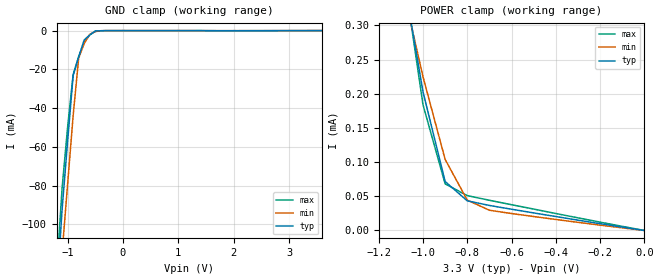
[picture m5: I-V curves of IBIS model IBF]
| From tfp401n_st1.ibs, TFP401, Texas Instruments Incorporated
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|   INPUT  MODEL WITH HYSTERESIS
[Model]   IBF
Model_type   Input
| Signals   STAG
Vinl = 1.08
Vinh = 2.10
| variable   typ   min   max
C_comp   2pF   NA   NA
|   typ   min   max
[Temperature Range] 25.0   70.0   0.0
[Voltage range]   3.3V   3.0V   3.6V
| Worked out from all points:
|   GND clamp passes 1 mA (typ) near -0.54 V on its own axis
|   POWER clamp passes 1 mA (typ) near -1.37 V on its own axis
[GND_clamp]
|Voltage   I(typ)   I(min)   I(max)
-3.6V     -1.31A     -1.33A     -1.29A
-1.2V     -138mA     -161mA     -126mA
-1.1V     -92.5mA    -115mA     -81.5mA
-1V       -57.2mA    -79.3mA    -49.9mA
-900mV    -23.2mA    -44mA      -22.7mA
-800mV    -13.6mA    -14.2mA    -13.4mA
-700mV    -4.78mA    -6.61mA    -6.2mA
-600mV    -2.27mA    -1.86mA    -2.19mA
-500mV    -190uA     -498uA     -401uA
-300mV    -547nA     -2.69uA    -1.84uA
3.6V      15.1uA     24.8uA     1.33nA
[Power_clamp]
|Note that the [Power_clamp] voltage table is referenced to Vcc
|and is calculated using Vtable=Vcc-Vmeasured.
|Voltage   I(typ)   I(min)   I(max)
-3.3V     5.57mA     4.01mA     6.85mA
-1.1V     392uA      367uA      405uA
-1V       203uA      225uA      184uA
-900mV    71.6uA     104uA      68.2uA
-800mV    43.4uA     44.4uA     51uA
-700mV    36.6uA     29.6uA     44.2uA
0V        35.3pA     99.7pA     34.3pA
